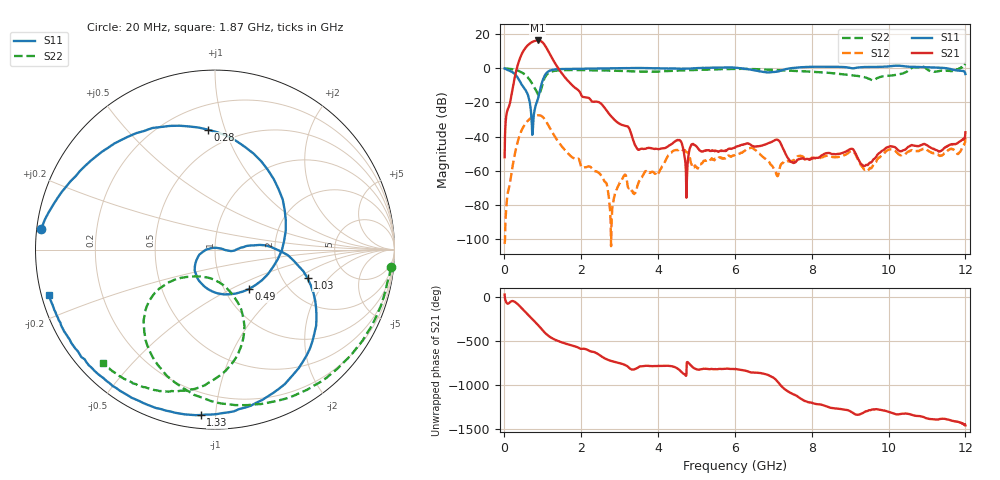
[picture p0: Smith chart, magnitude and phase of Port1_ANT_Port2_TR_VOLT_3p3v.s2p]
! Created Mon Aug 25 11:23:37 2025
# hz S ma R 50
! 2 Port Network Data from SP1.SP block
! freq  magS11  angS11  magS21  angS21  magS12  angS12  magS22  angS22
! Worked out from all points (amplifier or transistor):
!   1200 points, 10 MHz to 12 GHz, reference 50 ohm
!   highest |S21| = 16.3 dB at 870 MHz (marker M1)
!   |S21| within 3 dB of that: 604.5 MHz to 1.062 GHz (457.8 MHz wide, 54.9 % of centre)
!   unconditionally stable (mu >= 1): start of sweep to 2.671 GHz; 3.949 GHz to 4.971 GHz; 6.17 GHz to 7.451 GHz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
!   at 2.01 GHz: K = 42.34, MAG = 1.7 dB, |S12| = -58.0 dB
!   at 6.01 GHz: K = -236.14, MSG = 2.1 dB, |S12| = -50.6 dB
!   at 12 GHz: K = -1719.58, MSG = 1.5 dB, |S12| = -40.6 dB
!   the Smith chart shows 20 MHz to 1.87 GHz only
!   S11 on the Smith chart (normalised r, x): 20 MHz: 0.01, +0.06; 280 MHz: 0.36, +0.87; 490 MHz: 1.30, -0.62; 1.03 GHz: 2.73, -1.22; 1.33 GHz: 0.07, -0.91; 1.87 GHz: 0.02, -0.13
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1e7  0.9818 176.4  0.002477 28.8  7.229e-06 -132.2  0.99 -3.2
2e7  0.9743 173.1  0.0101 -14.0  9.301e-06 -132.9  0.985 -5.8
2.8e8  0.6694 93.4  0.5847 -56.0  0.003234 157.2  0.9024 -71.1
3.8e8  0.4699 36.6  1.573 -92.5  0.009138 118.4  0.8324 -93.9
4.9e8  0.2901 -49.2  3.084 -142.7  0.01844 67.6  0.7164 -116.5
5.8e8  0.2038 -111.6  4.299 176.3  0.02624 27.2  0.5894 -132.1
6.6e8  0.1063 -155.3  5.242 140.6  0.03248 -7.8  0.46 -142.3
7.7e8  0.04346 4.4  6.166 91.4  0.03898 -55.9  0.297 -143.9
8.7e8  0.1197 0.2  6.509 45.7  0.04199 -100.3  0.1791 -123.4
9.5e8  0.2798 4.9  6.233 6.6  0.04092 -138.2  0.2219 -73.4
1.03e9  0.5394 -17.2  5.196 -33.0  0.03465 -176.8  0.4569 -68.9
1.17e9  0.8312 -60.1  2.822 -88.2  0.01934 130.3  0.7445 -93.0
1.33e9  0.9251 -94.9  1.358 -127.7  0.009461 94.3  0.8468 -111.5
1.87e9  0.9573 -164.8  0.2545 153.7  0.002156 46.4  0.8851 -134.6
2.01e9  0.9604 -174.1  0.1593 129.5  0.001259 27.4  0.8847 -136.9
2.79e9  1.003 174.1  0.03825 -9.3  2.383e-05 106.8  0.8541 -148.7
4.01e9  0.9952 177.1  0.004299 -66.1  0.0008294 55.6  0.8007 142.0
6.01e9  1.035 145.8  0.004762 -99.6  0.00296 -42.0  0.9523 125.0
8.01e9  1.101 71.1  0.002294 -126.6  0.002396 -97.9  0.7873 141.6
1.001e10  1.136 -176.4  0.005038 130.2  0.004104 129.0  0.6021 103.7
1.099e10  1.068 -137.2  0.005674 58.3  0.004127 48.2  0.9603 66.4
1.2e10  0.6762 -71.4  0.01335 -23.8  0.009375 -50.9  1.339 -171.9
